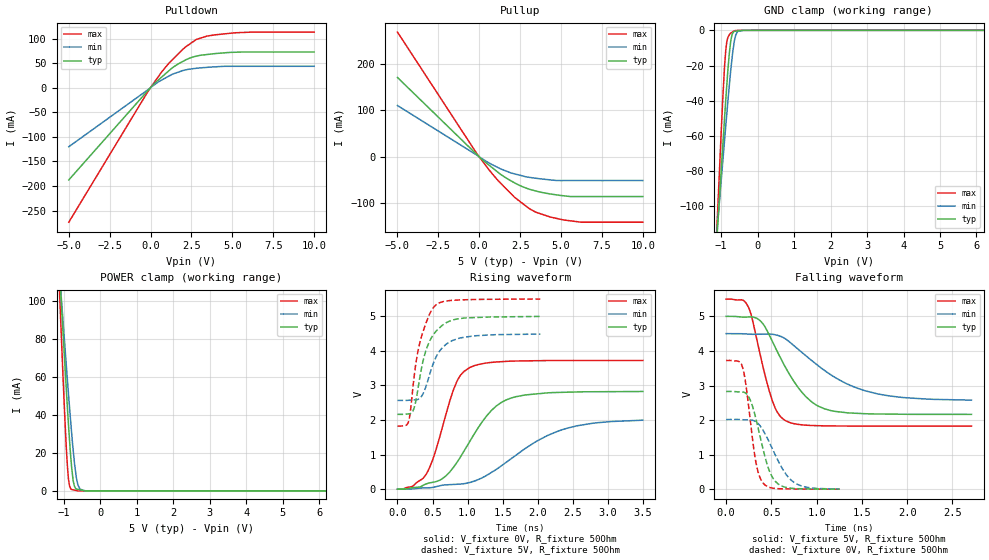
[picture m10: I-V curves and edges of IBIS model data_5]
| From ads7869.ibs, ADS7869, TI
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|   data_5 Model
[Model]   data_5
Model_type   I/O
Polarity   Non-Inverting
Enable   Active-Low
Vinl = 1.5
Vinh = 3.5
Vmeas = 2.5
Vref = 2.5
Cref = 30pF
Rref = 50
|   typ   min   max
|   (nom PVT)   (fast PVT)   (slow PVT)
|C_comp from frequency sweep method (F=8MHz)
|C_comp   3.350e-12   3.199e-12   3.470e-12
|ON state : BUFFER OUTPUT TURNED HIGH
|C_comp   3.715e-12   3.568e-12   3.796e-12
|OFF state: BUFFER OUTPUT TURNED LOW
|C_comp   2.948e-12   2.831e-12   3.143e-12
|C_comp from LC tank measurement(L=1nH)
|Resonant Frequency(Hz)   3.030e+09   3.070e+09   2.990e+09
C_comp   2.762e-12   2.690e-12   2.836e-12
|ON state : BUFFER OUTPUT TURNED HIGH
|Resonant Frequency(Hz)   3.030e+09   3.070e+09   2.990e+09
|C_comp   2.762e-12   2.690e-12   2.836e-12
|OFF state: BUFFER OUTPUT TURNED LOW
|Resonant Frequency(Hz)   2.980e+09   3.050e+09   2.840e+09
|C_comp   2.855e-12   2.726e-12   3.144e-12
| Where nom  PVT is Nominal Process, 5V, 36C
|   Fast PVT is Strong Process,  5.5V, -40C
|   Slow PVT is Weak Process,   4.5V, 96C
[Model Spec]
|Subparameter   typ   min   max
Vinh   3.5   3.15   3.85
Vinl   1.5   1.35   1.65
[Voltage Range]   5   4.5   5.5
|Ambient Temperature   25   85   -40
|Junction Temperature
[Temperature Range]   36   96   -40
[Pullup Reference]   5   4.5   5.5
[Pulldown Reference]   0   0   0
[Power Clamp Reference]   5   4.5   5.5
[GND Clamp Reference]   0   0   0
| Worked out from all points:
|   slope of the pulldown table from 0 to 0.75 V, typ, clamps not added: 31.7 ohm
|   slope of the pullup table from 0 to 0.75 V, typ, clamps not added: 33.6 ohm
|   GND clamp passes 1 mA (typ) near -0.67 V on its own axis
|   POWER clamp passes 1 mA (typ) near -0.66 V on its own axis
|   falling waveform, V_fixture 5V, R_fixture 50Ohm: 20-80 % time 380ps typ, 645ps min, 208ps max; typ from 5 V to 2.17 V
|   rising waveform, V_fixture 0V, R_fixture 50Ohm: 20-80 % time 561ps typ, 920ps min, 337ps max; typ from 0 V to 2.83 V
|   rising waveform, V_fixture 5V, R_fixture 50Ohm: 20-80 % time 220ps typ, 242ps min, 199ps max; typ from 2.16 V to 5 V
|   falling waveform, V_fixture 0V, R_fixture 50Ohm: 20-80 % time 166ps typ, 240ps min, 111ps max; typ from 2.83 V to 0.004 V
[Pulldown]
|   Voltage   I(typ)   I(min)   I(max)
-5V       -187.7mA   -120.2mA   -273.8mA
-180mV    -6.522mA   -4.696mA   -8.69mA
245mV     8.982mA    6.118mA    11.71mA
885mV     27.58mA    19.23mA    40.46mA
1.315V    40.07mA    27.03mA    56.05mA
2.167V    56.83mA    36.3mA     83.54mA
2.804V    64.08mA    39.51mA    98.2mA
3.448V    67.42mA    41.29mA    105mA
3.965V    69.32mA    42.4mA     107.6mA
5.159V    72.06mA    43.48mA    111.6mA
6.226V    72.49mA    43.48mA    113.1mA
10V       72.49mA    43.48mA    113.1mA
[GND Clamp]
|   Voltage   I(typ)   I(min)   I(max)
-5V       -1.398A    -1.087A    -1.912A
-1.247V   -160.9mA   -147mA     -171.9mA
-1.04V    -93.06mA   -95.47mA   -76.81mA
-952mV    -64.52mA   -73.65mA   -37.65mA
-908mV    -50.27mA   -62.74mA   -20.96mA
-875mV    -40.02mA   -54.61mA   -11.66mA
-814.5mV  -22.39mA   -40.13mA   -3.93mA
-740mV    -6.545mA   -23.33mA   -1.632mA
-649.5mV  -646.7uA   -7.684mA   -347.2uA
-549.5mV  -392.6uA   -698.7uA   -57.01uA
-396.5mV  -3.812uA   -4.517uA   -5.613uA
10V       0A         0A         0A
[Pullup]
|   Voltage   I(typ)   I(min)   I(max)
-5V       171.3mA    110.8mA    269.3mA
-180mV    5.912mA    4.327mA    8.552mA
245mV     -8.177mA   -5.651mA   -11.62mA
885mV     -26.12mA   -18.69mA   -40.46mA
1.315V    -38.17mA   -26.24mA   -57.25mA
2.188V    -56.89mA   -37.12mA   -88.42mA
3.091V    -70.33mA   -44.49mA   -112.6mA
3.448V    -73.73mA   -46.27mA   -119.5mA
4.361V    -80.33mA   -49.92mA   -130.3mA
5.159V    -84.2mA    -51.24mA   -136.4mA
6.226V    -85.87mA   -51.24mA   -141.2mA
10V       -85.87mA   -51.24mA   -141.2mA
[POWER Clamp]
|   Voltage   I(typ)   I(min)   I(max)
-5V       1.442A     1.134A     1.932A
-1.247V   160mA      148.3mA    165mA
-1.04V    89.52mA    94.08mA    68.54mA
-979.5mV  69.48mA    78.45mA    41.54mA
-902.5mV  44.12mA    58.61mA    13.25mA
-869.5mV  34.13mA    50.44mA    5.771mA
-798mV    15.25mA    33.33mA    822.7uA
-740mV    5.096mA    20.8mA     568.6uA
-653mV    976.5uA    6.559mA    187.6uA
-558.5mV  618.8uA    1.078mA    1.061uA
-468.5mV  278.2uA    251.4uA    890.1nA
10V       0A         0A         0A
[Ramp]
R_load = 50
|   typ   min   max
dV/dt_r   1.69522/5.60682e-10   1.19681/9.16281e-10   2.23403/3.37269e-10
dV/dt_f   1.70154/3.80036e-10   1.15855/6.50823e-10   2.20473/2.08222e-10
[Falling Waveform]
V_fixture = 5V
V_fixture_min = 4.5V
V_fixture_max = 5.5V
R_fixture = 50Ohm
|   Time   V(typ)   V(min)   V(max)
0s        5V         4.5V       5.5V
184.8ps   4.977V     4.496V     5.47V
243.5ps   4.982V     4.488V     5.28V
386.7ps   4.846V     4.484V     3.773V
515.3ps   4.25V      4.48V      2.524V
668ps     3.469V     4.326V     1.968V
878.6ps   2.683V     3.866V     1.854V
1.154ns   2.277V     3.316V     1.831V
1.743ns   2.175V     2.724V     1.826V
2.71ns    2.166V     2.578V     1.826V
[Rising Waveform]
V_fixture = 0V
V_fixture_min = 0V
V_fixture_max = 0V
R_fixture = 50Ohm
|   Time   V(typ)   V(min)   V(max)
0s        1.133nV    9.184nV    1.013nV
209.9ps   41.68mV    6.018mV    77.86mV
408.2ps   150.7mV    37.86mV    428.4mV
539.7ps   212.3mV    67.83mV    1.079V
807.7ps   656.3mV    137.6mV    2.922V
1.018ns   1.336V     186.7mV    3.502V
1.345ns   2.287V     489.7mV    3.668V
1.616ns   2.633V     873.2mV    3.703V
2.43ns    2.805V     1.768V     3.721V
3.5ns     2.825V     1.995V     3.723V
[Rising Waveform]
V_fixture = 5V
V_fixture_min = 4.5V
V_fixture_max = 5.5V
R_fixture = 50Ohm
|   Time   V(typ)   V(min)   V(max)
0s        2.164V     2.568V     1.825V
159.1ps   2.178V     2.571V     1.958V
184.8ps   2.188V     2.575V     2.253V
234.3ps   2.325V     2.581V     3.19V
307.6ps   3.09V      2.612V     4.136V
404.9ps   4.001V     2.959V     4.789V
539.7ps   4.542V     3.775V     5.312V
692.9ps   4.812V     4.189V     5.441V
905.7ps   4.939V     4.377V     5.475V
2.038ns   4.996V     4.485V     5.499V
[Falling Waveform]
V_fixture = 0V
V_fixture_min = 0V
V_fixture_max = 0V
R_fixture = 50Ohm
|   Time   V(typ)   V(min)   V(max)
0s        2.826V     2.017V     3.723V
134.3ps   2.816V     2.018V     3.702V
184.8ps   2.812V     2.011V     3.502V
253.6ps   2.655V     2.007V     2.289V
323.8ps   2.093V     1.962V     853.2mV
366.2ps   1.627V     1.862V     392.2mV
408.2ps   1.16V      1.704V     178.3mV
518.3ps   316.8mV    1.128V     30.72mV
720.6ps   29.92mV    258.1mV    8.95mV
1.253ns   4.275mV    7.74mV     2.68mV
